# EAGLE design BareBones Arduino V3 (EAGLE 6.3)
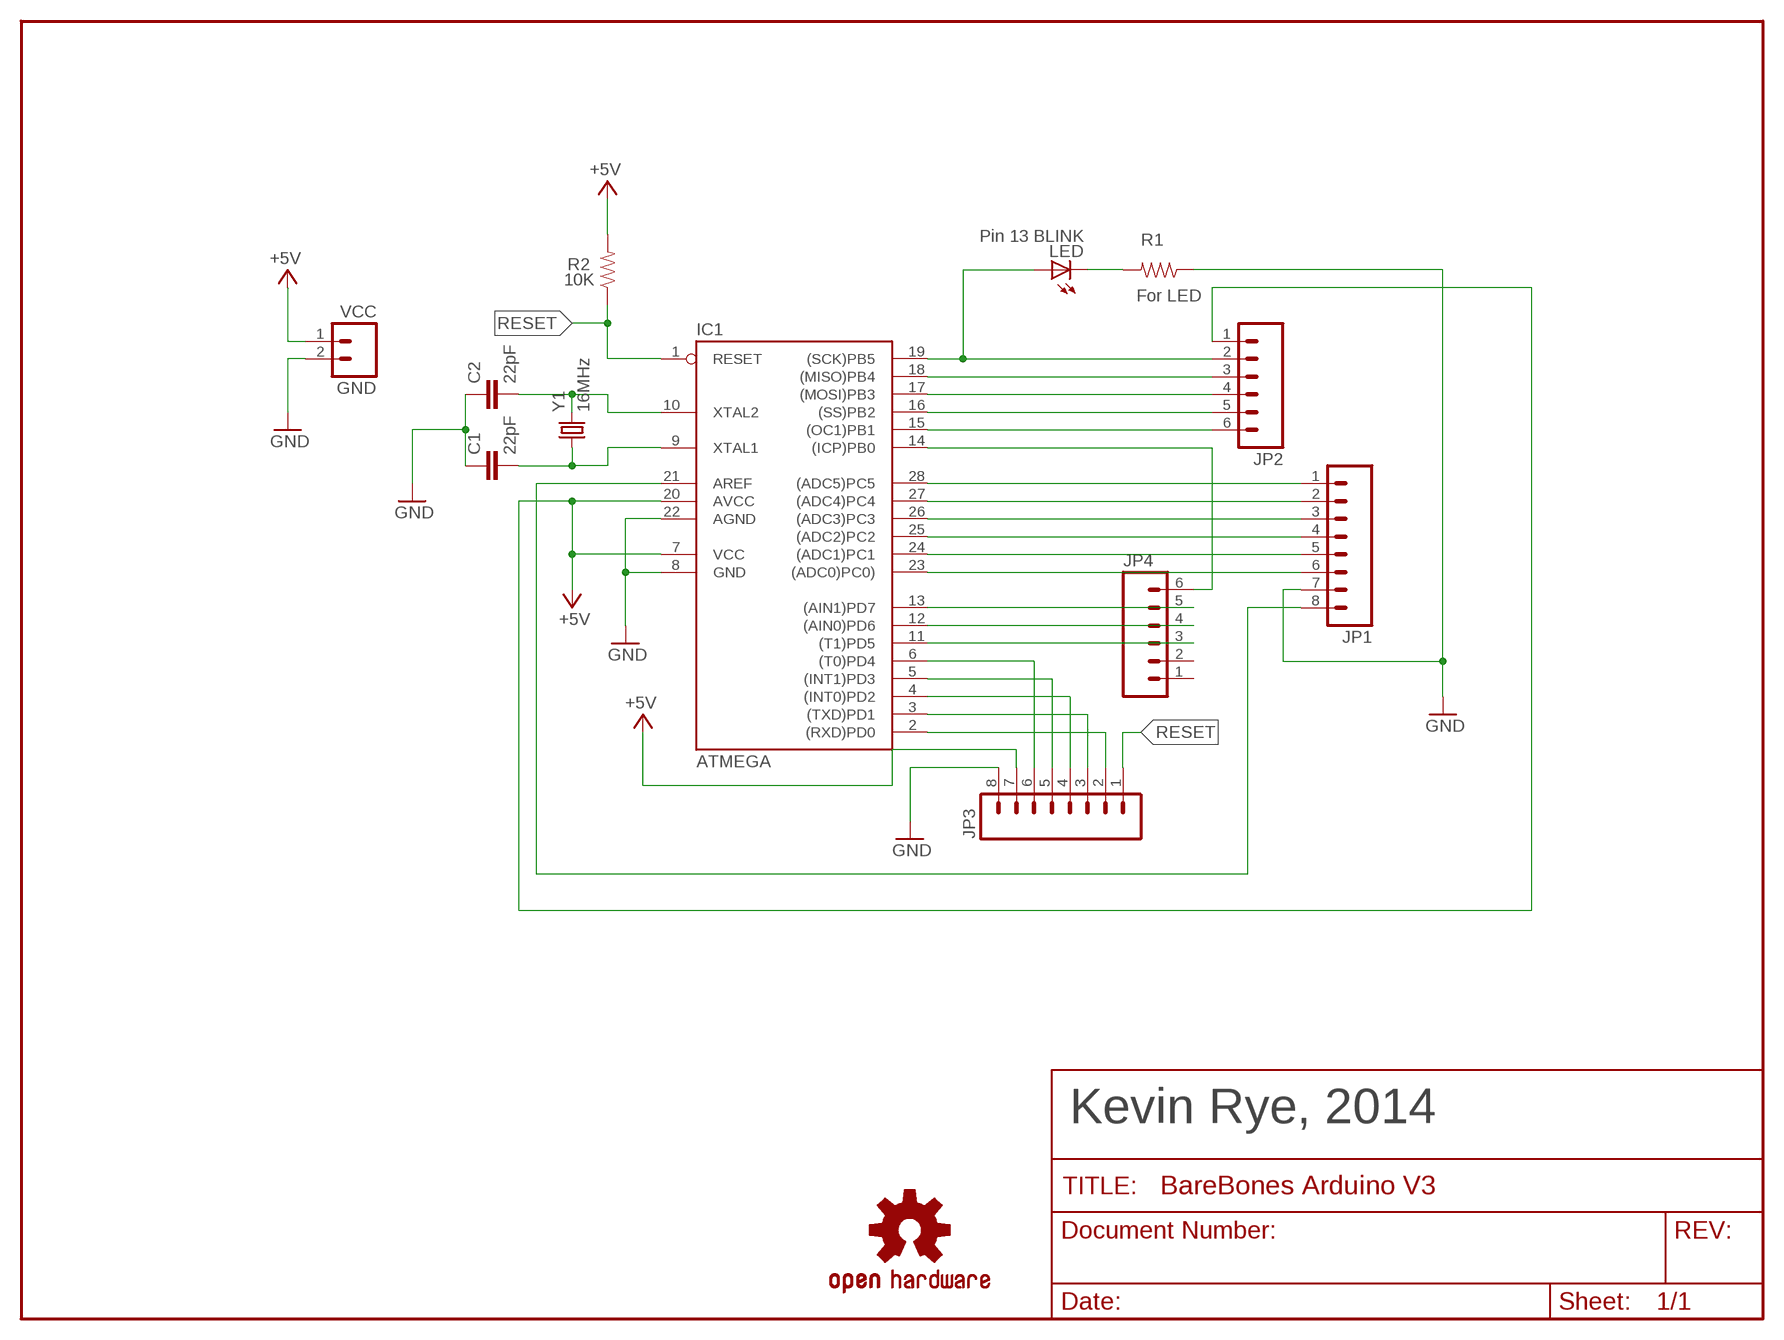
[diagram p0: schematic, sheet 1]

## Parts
C1  22pF  CAP0805  [0805]
C2  22pF  CAP0805  [0805]
GND  VCC  M02PTH  [1X02]
IC1  ATMEGA  AT90S4433P  [DIL28-3]
JP1  M081X08  [1X08]
JP2  M06SIP  [1X06]
JP3  M081X08  [1X08]
JP4  M06SIP  [1X06]
LED  Pin 13 BLINK  LED-GREEN0603  [LED-0603]
R1  For LED  RESISTOR0805-RES  [0805]
R2  10K  RESISTOR0805-RES  [0805]
U$1  OSHW-LOGOS  [OSHW-LOGO-S]
Y1  16MHz  CRYSTAL5X3  [CRYSTAL-SMD-5X3]

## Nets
+5V [power]: GND.1 IC1.7(VCC) IC1.20(AVCC) JP2.1 JP3.7 R2.2
GND [power]: C1.1 C2.1 GND.2 IC1.8(GND) IC1.22(AGND) JP1.7 JP3.8 R1.1
M8RXD: IC1.2((RXD)PD0) JP3.2
N$1: IC1.18((MISO)PB4) JP2.3
N$3: IC1.24((ADC1)PC1) JP1.5
N$4: IC1.17((MOSI)PB3) JP2.4
N$5: IC1.11((T1)PD5) JP4.3
N$6: C1.2 IC1.9(XTAL1) Y1.1
N$7: C2.2 IC1.10(XTAL2) Y1.3
N$8: LED.C R1.2
N$9: IC1.3((TXD)PD1) JP3.3
N$10: IC1.4((INT0)PD2) JP3.4
N$11: IC1.5((INT1)PD3) JP3.5
N$12: IC1.6((T0)PD4) JP3.6
N$13: IC1.12((AIN0)PD6) JP4.4
N$14: IC1.13((AIN1)PD7) JP4.5
N$15: IC1.14((ICP)PB0) JP4.6
N$16: IC1.15((OC1)PB1) JP2.6
N$17: IC1.16((SS)PB2) JP2.5
N$18: IC1.23((ADC0)PC0)) JP1.6
N$19: IC1.25((ADC2)PC2) JP1.4
N$20: IC1.26((ADC3)PC3) JP1.3
N$21: IC1.27((ADC4)PC4) JP1.2
N$22: IC1.28((ADC5)PC5) JP1.1
N$23: IC1.21(AREF) JP1.8
RESET: IC1.1(RESET) JP3.1 R2.1
SCK: IC1.19((SCK)PB5) JP2.2 LED.A
Unconnected: JP4.1 JP4.2

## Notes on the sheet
- Kevin Rye, 2014

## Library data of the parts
C1 C2 = SparkFun-Capacitors:CAP: Capacitor
GND = SparkFun:M02: Header 2
IC1 = atmel:AT90S4433: MICROCONTROLLER 4 Kbytes FLASH 128 bytes SRAM 256 bytes EEPROM UART 6-channel 10 bit ADC
JP1 JP3 = SparkFun:M08: Header 8 Standard 8-pin 0.1" header. Use with straight break away headers (SKU : PRT-00116), right angle break away headers (PRT-00553), swiss pins (PRT-00743), machine pins (PRT-00117), and female headers (PRT-00115).
JP2 JP4 = SparkFun:M06: Header 6 Standard 6-pin 0.1" header. Use with straight break away headers (SKU : PRT-00116), right angle break away headers (PRT-00553), swiss pins (PRT-00743), machine pins (PRT-00117), and female headers (PRT-00115). Molex polarized connector foot print use with SKU : PRT-08094 with associated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
LED = SparkFun-LED:LED-GREEN: Various green LEDs; PROD_ID: DIO-00821; VALUE: GREEN
R1 R2 = SparkFun-Resistors:RESISTOR: Resistor
U$1 = SparkFun:OSHW-LOGO: Open Source Hardware Logo This logo indicates the piece of hardware it is found on incorporates a OSHW license and/or adheres to the definition of open source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
Y1 = SparkFun-FreqCtrl:CRYSTAL: Various standard crystals. Proven footprints. Spark Fun Electronics SKU : COM-00534

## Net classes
0 default: width 0.4 mm, clearance 0.3 mm
1 power: width 0.6 mm, clearance 0.3 mm

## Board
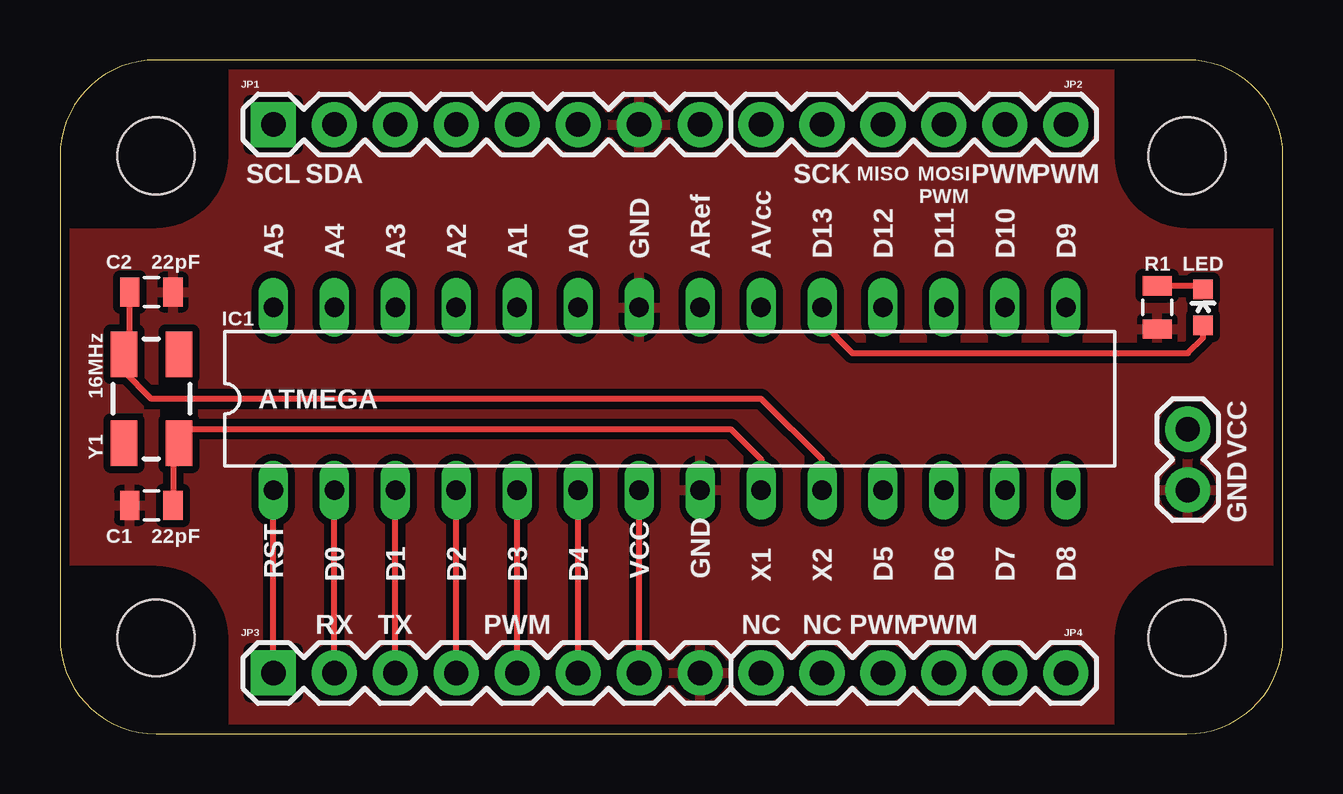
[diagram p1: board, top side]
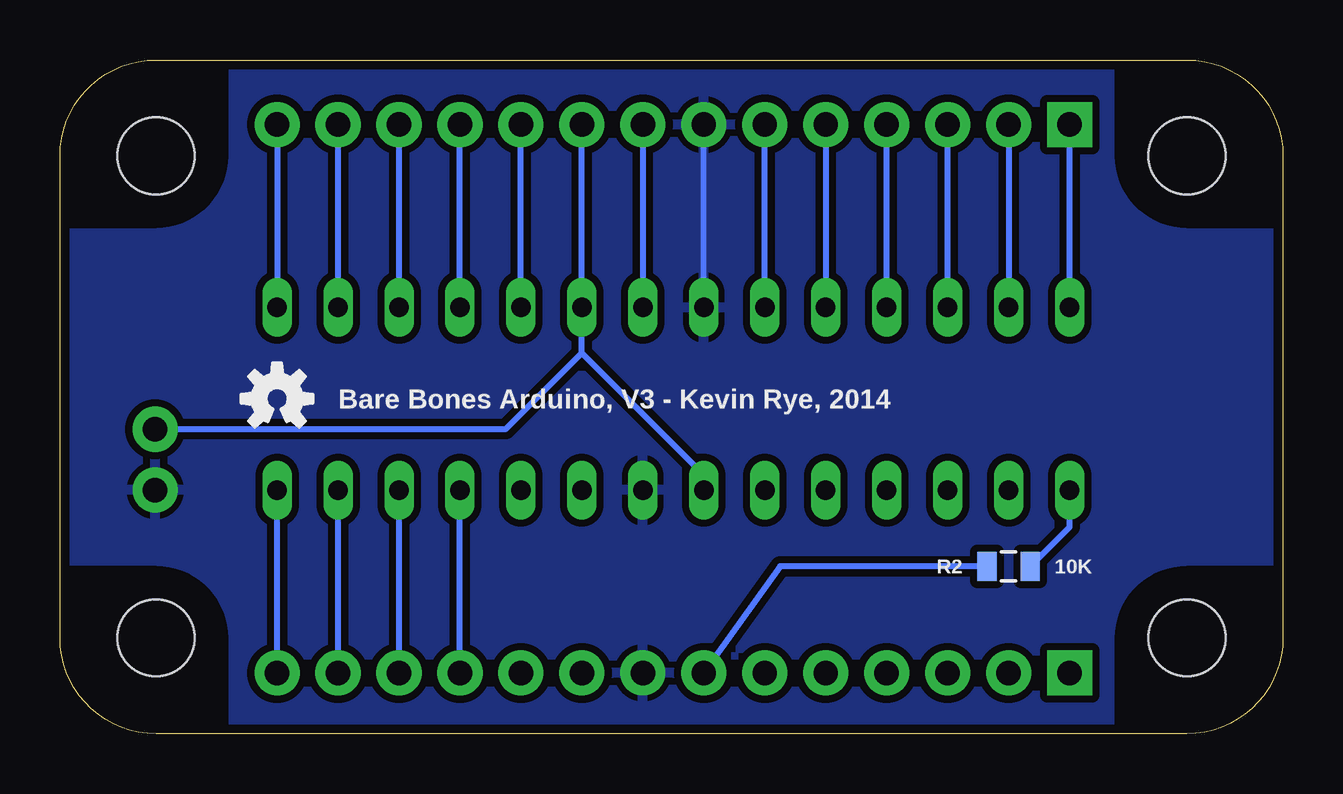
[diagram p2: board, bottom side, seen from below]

Size 50.95 x 28.09 mm. Coordinates in mm from the lower left corner, seen from the top.
Copper layers (1*16): Top 0.0356mm / dielectric 1.5011mm / Bottom 0.0356mm
Design rules "LaenPCBOrder": minimum track width 6mil, minimum drill 13mil, track to track 6mil, track to pad 6mil, pad to pad 6mil, via to via 6mil, smd to smd 6mil, copper to edge 15mil, drill to drill 6mil, minimum pad ring 7mil, minimum via ring 7mil, stop-mask expansion 3mil, vias tented up to drill 0mil, thermal gap 10mil

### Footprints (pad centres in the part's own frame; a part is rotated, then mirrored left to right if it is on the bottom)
0805 = smd 0.8 x 1.2: 1 -0.9,0; 2 0.9,0
1X02 = drill 1.016 pad 1.88: 1 0,0; 2 2.54,0
DIL28-3 = drill 0.813 long: 1 -16.51,-3.81; 2 -13.97,-3.81; 3 -11.43,-3.81; 4 -8.89,-3.81; 5 -6.35,-3.81; 6 -3.81,-3.81; 7 -1.27,-3.81; 8 1.27,-3.81; 9 3.81,-3.81; 10 6.35,-3.81; 11 8.89,-3.81; 12 11.43,-3.81; 13 13.97,-3.81; 14 16.51,-3.81; 15 16.51,3.81; 16 13.97,3.81; 17 11.43,3.81; 18 8.89,3.81; 19 6.35,3.81; 20 3.81,3.81; 21 1.27,3.81; 22 -1.27,3.81; 23 -3.81,3.81; 24 -6.35,3.81; 25 -8.89,3.81; 26 -11.43,3.81; 27 -13.97,3.81; 28 -16.51,3.81
1X08 = drill 1.016 pad 1.88 square: 1 0,0 | drill 1.016 pad 1.88: 2 2.54,0; 3 5.08,0; 4 7.62,0; 5 10.16,0; 6 12.7,0; 7 15.24,0; 8 17.78,0
1X06 = drill 1.016 pad 1.88: 1 0,0; 2 2.54,0; 3 5.08,0; 4 7.62,0; 5 10.16,0; 6 12.7,0
LED-0603 = smd 0.8 x 0.8: A 0,-0.75; C 0,0.75
2.2X1 = hole 3.2: 4,4; 46.955,4; 46.955,24.095; 4,24.095
CRYSTAL-SMD-5X3 = smd 1.9 x 1.1: 1 -1.85,-1.15; 2 1.85,-1.15; 3 1.85,1.15; 4 -1.85,1.15

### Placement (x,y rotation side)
C1  3.81,9.53 0 top
C2  3.81,18.41 180 top
GND  46.99,12.7 270 top
IC1  25.4,13.97 0 top
JP1  8.89,25.4 0 top
JP2  29.21,25.4 0 top
JP3  8.89,2.54 0 top
JP4  29.21,2.54 0 top
LED  47.62,17.78 0 top
R1  45.72,17.78 90 top
R2  11.43,6.99 180 bottom
U$1  41.91,13.97 0 bottom
U$2  [2.2X1]  0,0 0 top
Y1  3.81,13.97 90 top

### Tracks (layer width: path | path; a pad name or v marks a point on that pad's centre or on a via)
+5V
  Top 0.254: JP3.7 IC1.7
  Bottom 0.254: JP2.1 IC1.20 29.21,15.88 | R2.2 20.95,6.99 JP3.7 | IC1.7 24.13,10.79 29.21,15.88 | GND.1 32.38,12.7 29.21,15.88
GND
  Bottom 0.254: IC1.22 JP1.7
  pour Top: -10.16,29.21 57.15,29.21 57.15,-1.27 -10.16,-1.27
  pour Bottom: -10.16,29.21 55.25,29.84 55.25,-0.64 -10.16,-1.27
M8RXD
  Top 0.254: JP3.2 IC1.2
N$1
  Bottom 0.254: IC1.18 JP2.3
N$3
  Bottom 0.254: JP1.5 IC1.24
N$4
  Bottom 0.254: IC1.17 JP2.4
N$5
  Bottom 0.254: JP4.3 IC1.11
N$6
  Top 0.254: IC1.9 29.21,11.43 27.94,12.7 5.08,12.7 4.96,12.58 Y1.1 4.71,11.87 C1.2
N$7
  Top 0.254: 2.66,15.76 Y1.3 | IC1.10 31.75,11.43 29.21,13.97 3.81,13.97 2.66,15.12 Y1.3 | Y1.3 2.91,16.07 C2.2
N$8
  Top 0.254: R1.2 47.62,18.68 LED.C
N$9
  Top 0.254: JP3.3 IC1.3
N$10
  Top 0.254: JP3.4 IC1.4
N$11
  Top 0.254: JP3.5 IC1.5
N$12
  Top 0.254: JP3.6 IC1.6
N$13
  Bottom 0.254: JP4.4 IC1.12
N$14
  Bottom 0.254: JP4.5 IC1.13
N$15
  Bottom 0.254: JP4.6 IC1.14
N$16
  Bottom 0.254: JP2.6 IC1.15
N$17
  Bottom 0.254: IC1.16 JP2.5
N$18
  Bottom 0.254: IC1.23 JP1.6
N$19
  Bottom 0.254: IC1.25 JP1.4
N$20
  Bottom 0.254: IC1.26 JP1.3
N$21
  Bottom 0.254: JP1.2 IC1.27
N$22
  Bottom 0.254: IC1.28 JP1.1
N$23
  Bottom 0.254: JP1.8 IC1.21
RESET
  Top 0.254: JP3.1 IC1.1
  Bottom 0.254: R2.1 8.89,8.62 IC1.1
SCK
  Top 0.254: IC1.19 31.75,17.14 33.02,15.88 46.99,15.88 47.62,16.51 LED.A
  Bottom 0.254: IC1.19 JP2.2

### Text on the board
Unrouted: This work is licensed under a Creative Commons Attribution-NonCommercial-ShareAlike 4.0 International License. / http://creativecommons.org/licenses/by-nc-sa/4.0/deed.en_US
tNames: SCL | SDA | SCK | MISO | MOSI | PWM | PWM | PWM | C2 | 22pF | A5 | A4 | A3 | A2 | A1 | A0 | GND | ARef | AVcc | D13 | D12 | D11 | D10 | D9 | C1 | 22pF | RST | D0 | D1 | D2 | D3 | D4 | VCC | GND | X1 | X2 | D5 | D6 | D7 | D8 | RX | TX | PWM | NC | NC | PWM | PWM
bNames: Bare Bones Arduino, V3 - Kevin Rye, 2014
